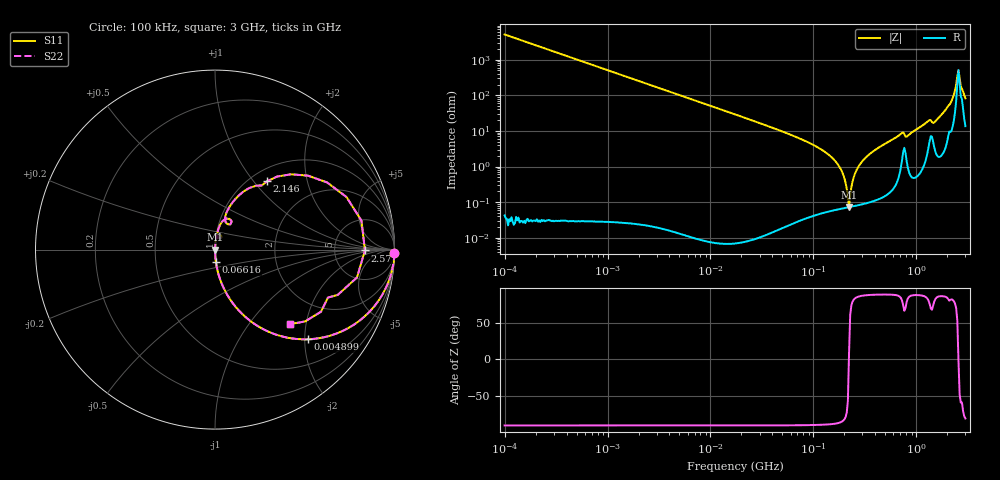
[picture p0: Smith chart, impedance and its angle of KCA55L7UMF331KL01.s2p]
!Murata Part Number: KCA55L7UMF331KL01
!These Parameters are Measured in Series Mode Connection
!Data Generated on Jan 08, 2026
!  o--ll--o
!Port1  Port2
!  o------o
!Operation Temp=25[degC], DC Bias Voltage=0[V]
!Freq. Start=100[kHz] Stop=3[GHz] 401[Steps]
# Hz S RI R 50
!Freq.(Hz) S11(Real) S11(Imag) S21(Real) S21(Imag) S12(Real) S12(Imag) S22(Real) S22(Imag)
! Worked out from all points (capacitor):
!   401 points, 100 kHz to 3 GHz, reference 50 ohm
!   read as one part in series: C = 314 pF near 105.3 kHz
!   lowest |Z| = 73.3 mohm at 222.2 MHz (marker M1)
!   series resonance near 221.6 MHz, so ESL is about 1.6 nH
!   S11 on the Smith chart (normalised r, x): 100 kHz: open; 4.899 MHz: 1.00, -2.07; 66.16 MHz: 1.00, -0.14; 2.146 GHz: 1.19, +1.17; 2.57 GHz: 11, -0; 3 GHz: 1.27, -1.62
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100000  0.9996 -0.0197  0.000388 0.0197  0.000388 0.0197  0.9996 -0.0197
562235  0.9879 -0.1094  0.0121 0.1094  0.0121 0.1094  0.9879 -0.1094
3161081  0.7204 -0.4487  0.2796 0.4487  0.2796 0.4487  0.7204 -0.4487
4899066  0.5175 -0.4996  0.4825 0.4996  0.4825 0.4996  0.5175 -0.4996
1.77727e7  0.0746 -0.2625  0.9254 0.2625  0.9254 0.2625  0.0746 -0.2625
6.615861e7  0.0051 -0.0693  0.9949 0.0693  0.9949 0.0693  0.0051 -0.0693
9.738194e7  0.00215 -0.0418  0.9978 0.0418  0.9978 0.0418  0.00215 -0.0418
1.716802e8  0.00076 -0.0118  0.9992 0.0118  0.9992 0.0118  0.00076 -0.0118
1.952919e8  0.000705 -0.0058  0.9993 0.0058  0.9993 0.0058  0.000705 -0.0058
2.109903e8  0.000708 -0.00225  0.9993 0.00225  0.9993 0.00225  0.000708 -0.00225
2.221509e8  0.000724 0.00011  0.9993 -0.00011  0.9993 -0.00011  0.000724 0.00011
2.52704e8  0.000818 0.00605  0.9992 -0.00605  0.9992 -0.00605  0.000818 0.00605
2.874592e8  0.000996 0.0121  0.999 -0.0121  0.999 -0.0121  0.000996 0.0121
5.475153e8  0.00439 0.0507  0.9956 -0.0507  0.9956 -0.0507  0.00439 0.0507
8.269535e8  0.0144 0.0709  0.9856 -0.0709  0.9856 -0.0709  0.0144 0.0709
1.281618e9  0.0524 0.1671  0.9476 -0.1671  0.9476 -0.1671  0.0524 0.1671
1.495945e9  0.0584 0.1548  0.9416 -0.1548  0.9416 -0.1548  0.0584 0.1548
2.145926e9  0.2889 0.3803  0.7111 -0.3803  0.7111 -0.3803  0.2889 0.3803
2.378954e9  0.6251 0.3739  0.3749 -0.3739  0.3749 -0.3739  0.6251 0.3739
2.570185e9  0.8355 -0.00462  0.1645 0.00462  0.1645 0.00462  0.8355 -0.00462
2.776789e9  0.6293 -0.2673  0.3707 0.2673  0.3707 0.2673  0.6293 -0.2673
3e9  0.4153 -0.4161  0.5847 0.4161  0.5847 0.4161  0.4153 -0.4161
